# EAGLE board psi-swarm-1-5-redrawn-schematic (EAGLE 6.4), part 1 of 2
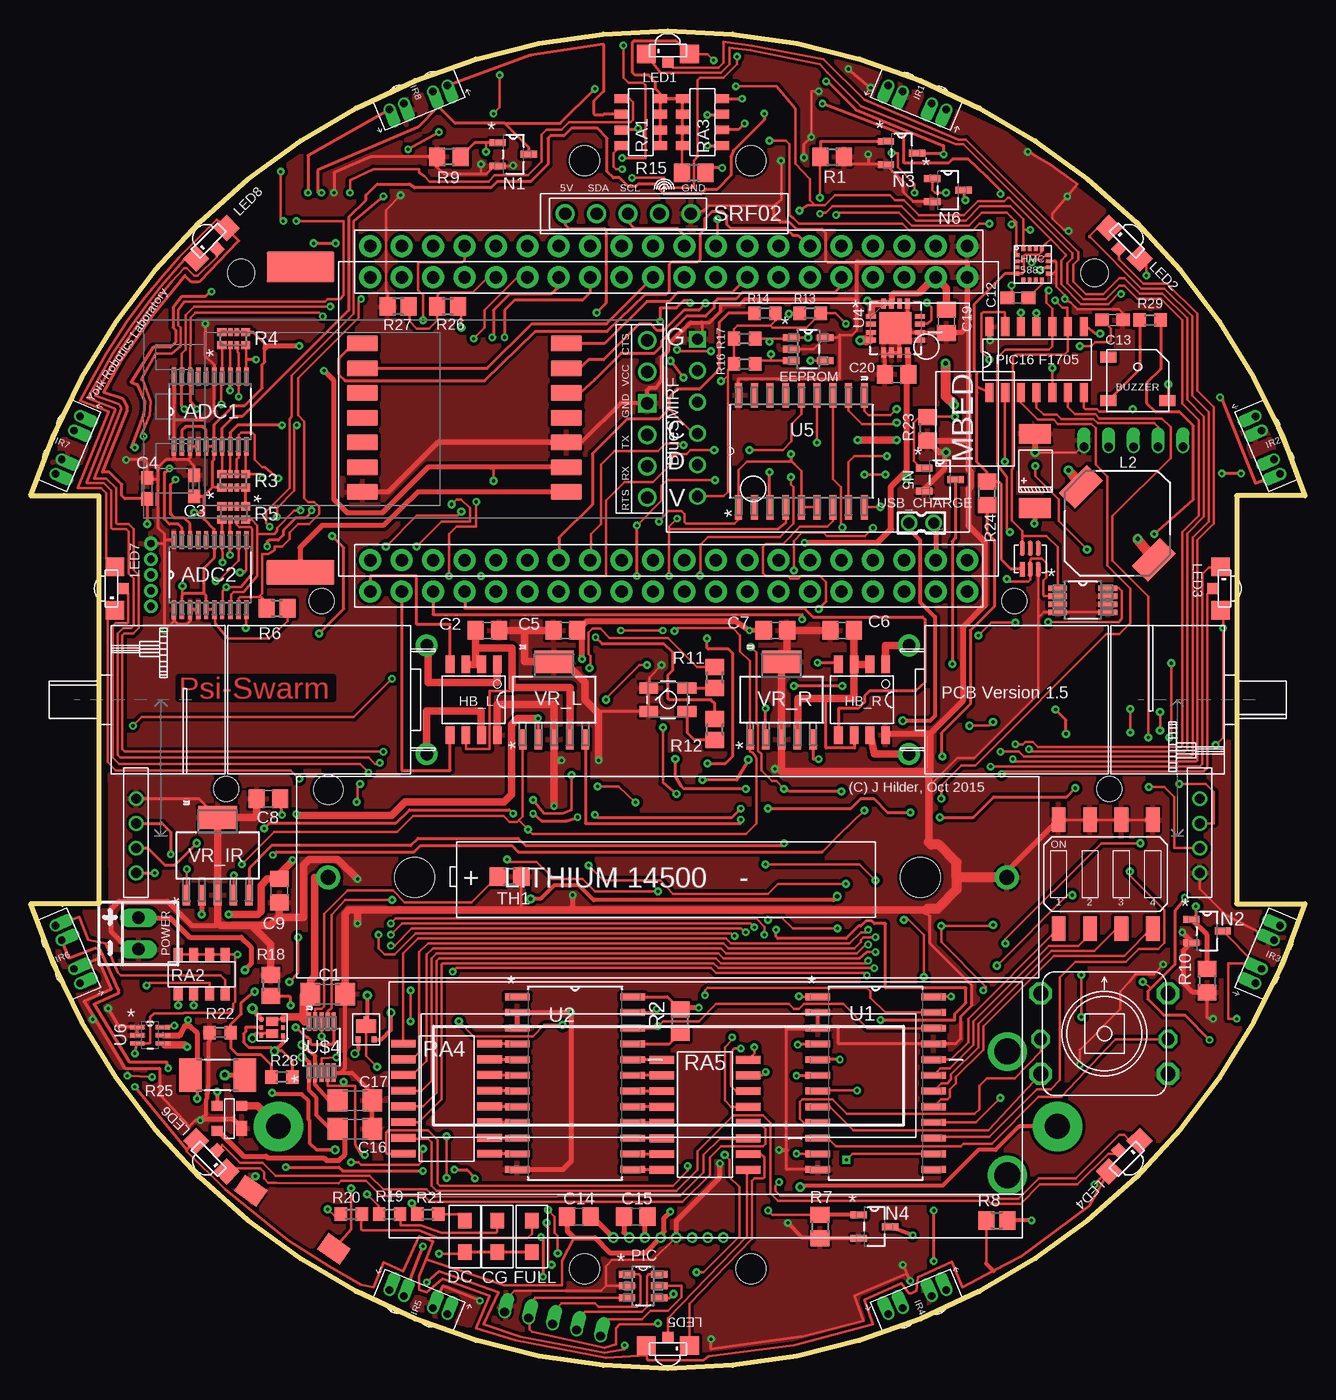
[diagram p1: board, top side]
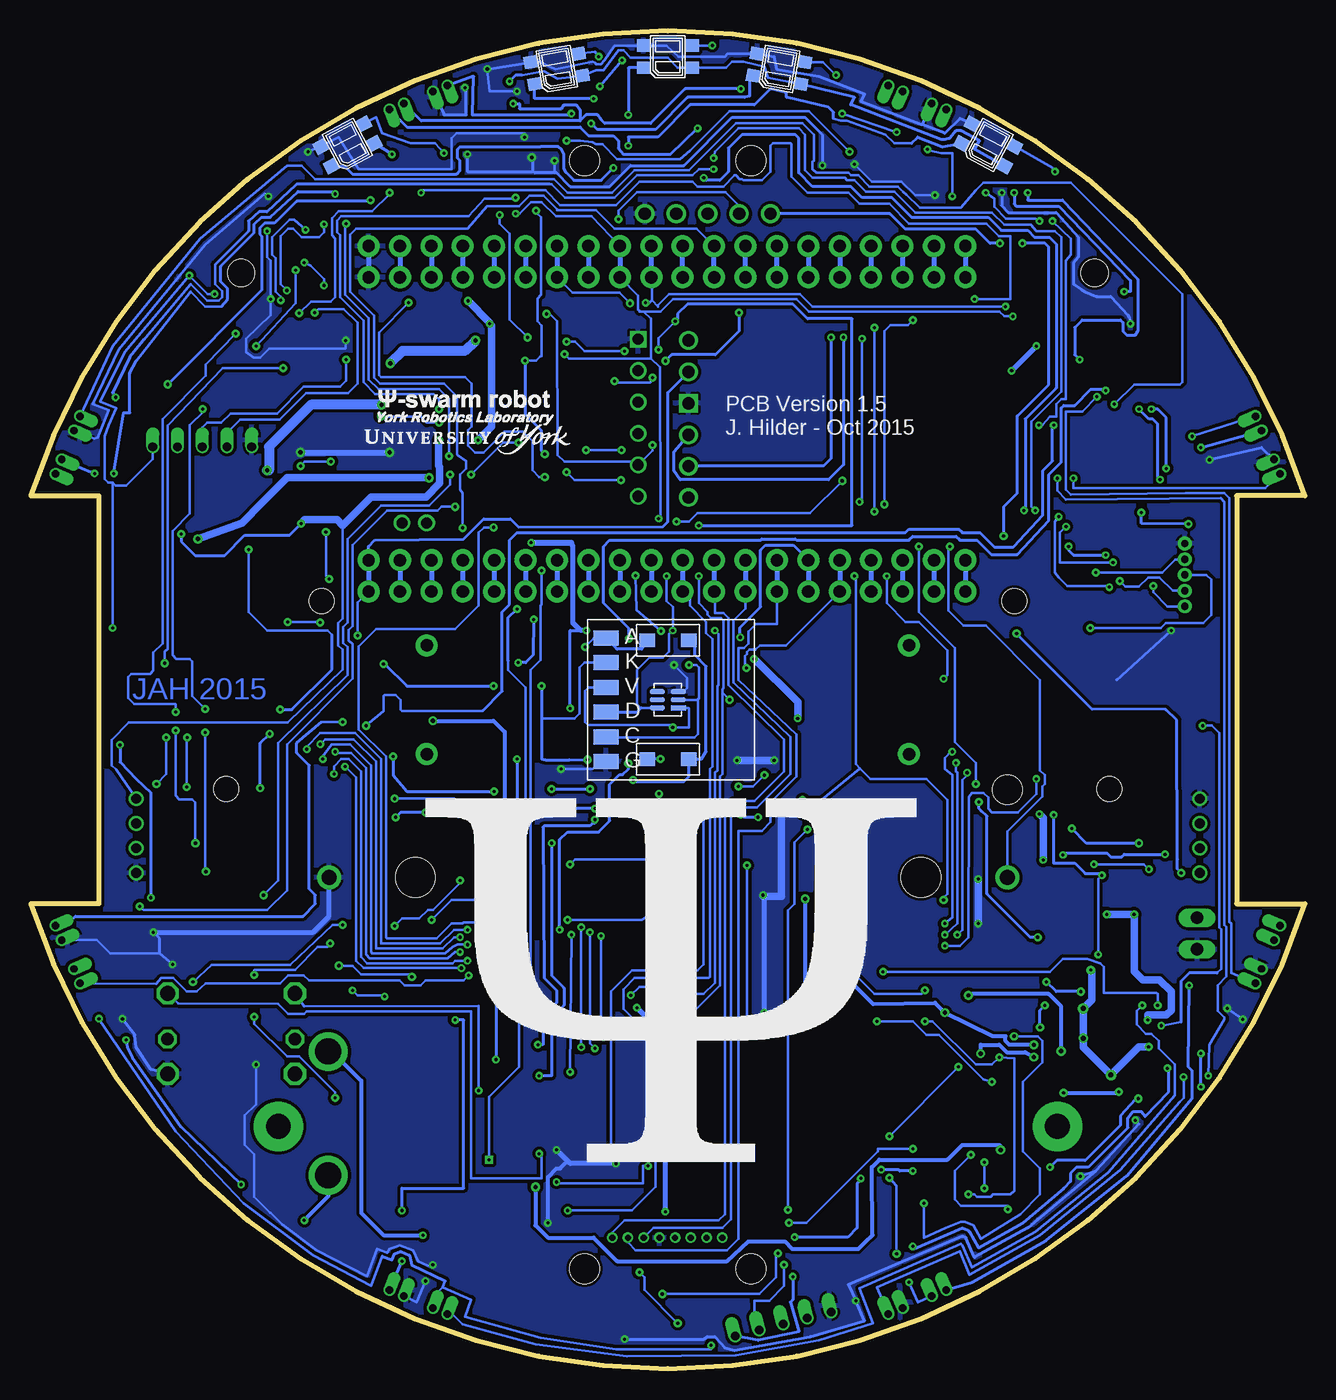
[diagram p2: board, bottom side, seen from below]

Size 103 x 108.16 mm. Coordinates in mm from the lower left corner, seen from the top.
Outline: 0,70.58 arc-144 103,70.58 97.5,70.58 97.5,37.58 103,37.58 arc-144 0,37.58 5.5,37.58 5.5,70.58 0,70.58
Copper layers (1*16): Top 0.018mm / dielectric 1.55mm / Bottom 0.018mm
Design rules "eC_2Layer_PClass6_BaseCopperO18_eCDefault *": minimum track width 0.15mm, minimum drill 0.25mm, track to track 0.15mm, track to pad 0.15mm, pad to pad 0.15mm, via to via 0.15mm, smd to smd 0mil, copper to edge 0.25mm, drill to drill 0.25mm, minimum pad ring 0.175mm, minimum via ring 0.125mm, stop-mask expansion 0mil, vias tented up to drill 0.45mm, thermal gap 0.2mm
Holes 2.4 mm at 44.77,97.68 58.23,97.68 44.77,8.08 58.23,8.08
Holes 2.2 mm at 17,88.58 86,88.58
Holes 2 mm at 23.5,62.08 79.5,62.08 15.8,46.88 87.2,46.88

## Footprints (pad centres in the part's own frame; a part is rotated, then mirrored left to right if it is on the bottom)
SOP65P640X120-20N = smd 1.473 x 0.356: 1 -2.819,2.921; 2 -2.819,2.286; 3 -2.819,1.626; 4 -2.819,0.965; 5 -2.819,0.33; 6 -2.819,-0.33; 7 -2.819,-0.965; 8 -2.819,-1.626; 9 -2.819,-2.286; 10 -2.819,-2.921; 11 2.819,-2.921; 12 2.819,-2.286; 13 2.819,-1.626; 14 2.819,-0.965; 15 2.819,-0.33; 16 2.819,0.33; 17 2.819,0.965; 18 2.819,1.626; 19 2.819,2.286; 20 2.819,2.921
C1206 = smd 1.6 x 1.8: 1 -1.4,0; 2 1.4,0
C0805 = smd 1.3 x 1.5: 1 -0.95,0; 2 0.95,0
C0603 = smd 1.1 x 1: 1 -0.85,0; 2 0.85,0
2917TANTALUM = smd 1.6 x 2.6: ANODE -3,0; CATHODE 3,0
SOT95P270X145-5N = smd 1.321 x 0.559: 1 -1.372,0.94; 2 -1.372,0; 3 -1.372,-0.94; 4 1.372,-0.94; 5 1.372,0.94
ROHM-BD6211 = smd 0.7 x 1.4: P$1 -1.905,-2.857; P$2 -0.635,-2.857; P$3 0.635,-2.857; P$4 1.905,-2.857; P$5 1.905,2.857; P$6 0.635,2.857; P$7 -0.635,2.857; P$8 -1.905,2.857
TCRT-1000 = drill 0.6 pad 1.016 offset: ANODE -2.54,1.2; CATHODE -1.27,1.2; COLLECTOR 2.54,1.2; EMITTER 1.27,1.2
QRE1113GR-1471020 = smd 1.1 x 1: P1-ANODE -1.95,-0.9; P2-CATHODE 1.95,-0.9; P3-COLLECTOR 1.95,0.9; P4-EMITTER -1.95,0.9
IND_ELL8TP = smd 1.8 x 3.2 rotated 45: 1 -2.95,-2.95; 2 2.95,2.95
KINGBRIGHT-KPBA3010 = smd 1.5 x 1.5: P1-ANODE -1.75,1.8; P3-CGREEN 1.75,1.8 | smd 0.9 x 0.9: P2-CRED 0,2.45
2322113-DUAL-LED-WURTH1411 = smd 1.5 x 0.9: 1 1.55,0.95; 2 1.55,-0.95; 3 -1.55,0.95; 4 -1.55,-0.95
01-ROBOT_LED-SMD = smd 1.25 x 1.1: AN -1.675,0; CA 1.675,0
MICROMETALGEARMOTOR = drill 1 pad 1.778: MOTOR+ 25.5,4.4; MOTOR- 25.5,-4.4
01-ROBOT_SOT95P280X130-3N = smd 1.321 x 0.559: 1 -1.27,0.94; 2 -1.27,-0.94; 3 1.27,0
01-ROBOT_SOT95P270X145-6N = smd 1.321 x 0.559: 1 -1.295,0.94; 2 -1.295,0; 3 -1.295,-0.94; 4 1.295,-0.94; 5 1.295,0; 6 1.295,0.94
22-23-2021 = drill 1 long: 1 -1.27,0; 2 1.27,0
R0805 = smd 1.3 x 1.5: 1 -0.95,0; 2 0.95,0
RESCAXE50P210X110X45-8N = smd 0.66 x 0.762: 1 -0.533,0.965; 4 -0.533,-0.965; 5 0.533,-0.965; 8 0.533,0.965 | smd 0.66 x 0.356: 2 -0.533,0.254; 3 -0.533,-0.254; 6 0.533,-0.254; 7 0.533,0.254
R0805' = smd 1.3 x 1.5: 1 -0.85,0; 2 0.85,0
R0603 = smd 1 x 1.1: 1 -0.85,0; 2 0.85,0
R2010 = smd 1.8 x 2.7: 1 -2.2,0; 2 2.2,0
VISHAY-CRA12E083-RES_ARRAY = smd 0.72 x 1.05: 1A 0,-1.6; 1B 0,1.6; 2A 1.27,-1.6; 2B 1.27,1.6; 3A 2.54,-1.6; 3B 2.54,1.6; 4A 3.81,-1.6; 4B 3.81,1.6
BOURNS-4816P = smd 2 x 0.63: 1 -3.493,0; 2 -3.493,-1.27; 3 -3.493,-2.54; 4 -3.493,-3.81; 5 -3.493,-5.08; 6 -3.493,-6.35; 7 -3.493,-7.62; 8 -3.493,-8.89; 9 3.493,-8.89; 10 3.493,-7.62; 11 3.493,-6.35; 12 3.493,-5.08; 13 3.493,-3.81; 14 3.493,-2.54; 15 3.493,-1.27; 16 3.493,0
ALPS-SKQUCAA010 = drill 1.2 octagon: P1 -5.15,3.25; P3 -5.15,-3.25; P4 5.15,-3.25; P6 5.15,3.25 | drill 1 octagon: P2 -5.15,-0.45; P5 5.15,-0.45
4WAYDIL-MCEMR-04-T = smd 1.1 x 2: 1 -3.81,-4.4; 2 -1.27,-4.4; 3 1.27,-4.4; 4 3.81,-4.4; 5 3.81,4.4; 6 1.27,4.4; 7 -1.27,4.4; 8 -3.81,4.4
SWITCH-1703878 = smd 2.2 x 1.6: 1 0,0; 2 8.2,0
01-ROBOT_SOIC127P1030X265-24N = smd 1.981 x 0.559: 1 -4.674,6.985; 2 -4.674,5.715; 3 -4.674,4.445; 4 -4.674,3.175; 5 -4.674,1.905; 6 -4.674,0.635; 7 -4.674,-0.635; 8 -4.674,-1.905; 9 -4.674,-3.175; 10 -4.674,-4.445; 11 -4.674,-5.715; 12 -4.674,-6.985; 13 4.674,-6.985; 14 4.674,-5.715; 15 4.674,-4.445; 16 4.674,-3.175; 17 4.674,-1.905; 18 4.674,-0.635; 19 4.674,0.635; 20 4.674,1.905; 21 4.674,3.175; 22 4.674,4.445; 23 4.674,5.715; 24 4.674,6.985
QFN65P400X400X100-17N = smd 0.813 x 0.381: 1 -1.981,0.965; 2 -1.981,0.33; 3 -1.981,-0.33; 4 -1.981,-0.965; 9 1.981,-0.965; 10 1.981,-0.33; 11 1.981,0.33; 12 1.981,0.965 | smd 0.381 x 0.813: 5 -0.965,-1.981; 6 -0.33,-1.981; 7 0.33,-1.981; 8 0.965,-1.981; 13 0.965,1.981; 14 0.33,1.981; 15 -0.33,1.981; 16 -0.965,1.981 | smd 2.591 x 2.591: 17 0,0
01-ROBOT_SOIC127P1030X265-18N = smd 1.981 x 0.559: 1 -4.521,5.08; 2 -4.521,3.81; 3 -4.521,2.54; 4 -4.521,1.27; 5 -4.521,0; 6 -4.521,-1.27; 7 -4.521,-2.54; 8 -4.521,-3.81; 9 -4.521,-5.08; 10 4.521,-5.08; 11 4.521,-3.81; 12 4.521,-2.54; 13 4.521,-1.27; 14 4.521,0; 15 4.521,1.27; 16 4.521,2.54; 17 4.521,3.81; 18 4.521,5.08
4WHEEL_ROBOT_LIBRARY_SOT65P210X110-6N = smd 1.168 x 0.356: 1 -1.041,0.66; 2 -1.041,0; 3 -1.041,-0.66; 4 1.041,-0.66; 5 1.041,0; 6 1.041,0.66
01-ROBOT_MBED-DUALSOCKET = drill 1 pad 1.778: P$1 0,0; P$2 0,-2.54; P$3 0,-5.08; P$4 0,-7.62; P$5 0,-10.16; P$6 0,-12.7; P$7 0,-15.24; P$8 0,-17.78; P$9 0,-20.32; P$10 0,-22.86; P$11 0,-25.4; P$12 0,-27.94; P$13 0,-30.48; P$14 0,-33.02; P$15 0,-35.56; P$16 0,-38.1; P$17 0,-40.64; P$18 0,-43.18; P$19 0,-45.72; P$20 0,-48.26; P$21 22.86,-48.26; P$22 22.86,-45.72; P$23 22.86,-43.18; P$24 22.86,-40.64; P$25 22.86,-38.1; P$26 22.86,-35.56; P$27 22.86,-33.02; P$28 22.86,-30.48; P$29 22.86,-27.94; P$30 22.86,-25.4; P$31 22.86,-22.86; P$32 22.86,-20.32; P$33 22.86,-17.78; P$34 22.86,-15.24; P$35 22.86,-12.7; P$36 22.86,-10.16; P$37 22.86,-7.62; P$38 22.86,-5.08; P$39 22.86,-2.54; P$40 22.86,0; P$41 -2.54,0; P$42 -2.54,-2.54; P$43 -2.54,-5.08; P$44 -2.54,-7.62; P$45 -2.54,-10.16; P$46 -2.54,-12.7; P$47 -2.54,-15.24; P$48 -2.54,-17.78; P$49 -2.54,-20.32; P$50 -2.54,-22.86; P$51 -2.54,-25.4; P$52 -2.54,-27.94; P$53 -2.54,-30.48; P$54 -2.54,-33.02; P$55 -2.54,-35.56; P$56 -2.54,-38.1; P$57 -2.54,-40.64; P$58 -2.54,-43.18; P$59 -2.54,-45.72; P$60 -2.54,-48.26; P$61 25.4,-48.26; P$62 25.4,-45.72; P$63 25.4,-43.18; P$64 25.4,-40.64; P$65 25.4,-38.1; P$66 25.4,-35.56; P$67 25.4,-33.02; P$68 25.4,-30.48; P$69 25.4,-27.94; P$70 25.4,-25.4; P$71 25.4,-22.86; P$72 25.4,-20.32; P$73 25.4,-17.78; P$74 25.4,-15.24; P$75 25.4,-12.7; P$76 25.4,-10.16; P$77 25.4,-7.62; P$78 25.4,-5.08; P$79 25.4,-2.54; P$80 25.4,0
KEYSTONE-1028-AAHOLDER = drill 1.2 pad 1.93: + 2.54,8.13; - 57.4,8.13 | hole 3.2: 9.53,8.13; 50.41,8.13 | hole 2.38: 2.54,15.22
01-ROBOT_MIDAS-MCCOG21605B6W-DISPLAY = drill 0.5: 1-VOUT 18.155,0; 2-CAPN 19.425,0; 3-CAPP 20.695,0; 4-VDD 21.965,0; 5-VSS 23.235,0; 6-SDA 24.505,0; 7-SCL 25.775,0; 8-RST 27.045,0 | drill 2.1: LED-A 50,5.05; LED-K 50,15.05
01-ROBOT_SOP50P490X110-8N = smd 1.499 x 0.33: 1 -2.057,0.991; 2 -2.057,0.508; 3 -2.057,0; 4 -2.057,-0.508; 5 -2.057,-0.991; 6 2.057,-0.991; 7 2.057,-0.508; 8 2.057,0; 9 2.057,0.508; 10 2.057,0.991
HMC5883L = smd 0.45 x 0.3: P$1 -1.3,0.75; P$2 -1.3,0.25; P$3 -1.3,-0.25; P$4 -1.3,-0.75; P$9 1.3,-0.75; P$10 1.3,-0.25; P$11 1.3,0.25; P$12 1.3,0.75 | smd 0.3 x 0.45: P$5 -0.75,-1.3; P$6 -0.25,-1.3; P$7 0.25,-1.3; P$8 0.75,-1.3; P$13 0.75,1.3; P$14 0.25,1.3; P$15 -0.25,1.3; P$16 -0.75,1.3
POLOLU_LIBRARY_ALPHA433 = smd 1.3 x 2.5: 1-SDO 0,0; 2-NIRQ 2,0; 3-FSK 4,0; 4-DCLK 6,0; 5-CLK 8,0; 6-NRES 10,0; 7-GND 12,0; 8-ANT 12,16.5; 9-VDD 10,16.5; 10-GND 8,16.5; 11-NINT 6,16.5; 12-SDI 4,16.5; 13-SCLK 2,16.5; 14-NSEL 0,16.5
NEW_PSISWARM_LIBRARY_PIC16F1705 = smd 0.65 x 1.55: P$1 0,-2.667; P$2 1.27,-2.667; P$3 2.54,-2.667; P$4 3.81,-2.667; P$5 5.08,-2.667; P$6 6.35,-2.667; P$7 7.62,-2.667; P$8 7.62,2.667; P$9 6.35,2.667; P$10 5.08,2.667; P$11 3.81,2.667; P$12 2.54,2.667; P$13 1.27,2.667; P$14 0,2.667
POLOLU_LIBRARY_2148530-433MHZANTENNA = smd 5.5 x 2: ANT 0,0 | smd 5.5 x 2.5: NC 0,24.7
NEW_PSISWARM_LIBRARY_SRF02-MODULE = drill 1 pad 1.55: 1-5V 0,0; 2-SDA 2.54,0; 3-SCL 5.08,0; 4-NC 7.62,0; 5-GND 10.16,0
01-ROBOT_BLUESMIRF-MODULE = drill 1: CTS -1.27,6.35; RTS -1.27,-6.35; RX -1.27,-3.81; TX -1.27,-1.27; VCC -1.27,3.81 | drill 1 square: GND -1.27,1.27
01-ROBOT_PMEG2020CPA-CCDIODE-1859909 = smd 0.4 x 0.5: P$1 -0.65,1.05; P$2 0.65,1.05 | smd 1.6 x 1.1: P$3 0,0 | smd 0.4 x 0.25: P$4 0,-0.675
EXPORTED_LIBRARYPSI-SWARM-V13_01-ROBOT_LED-SMD = smd 1.25 x 1.1: AN -1.275,0; CA 1.275,0
2191755-PMFPB8032XP-MOSFET-SCHOTTKY = smd 0.35 x 0.3: 1 -0.65,-0.875; 2 0,-0.875; 3 0.65,-0.875; 4 0.65,0.875; 5 0,0.875; 6 -0.65,0.875 | smd 0.7 x 1: 7 -0.49,0; 8 0.49,0
EXPORTED_LIBRARYPSI-SWARM-V13_01-ROBOT_P-TERMINALS = drill 2 pad 4: P$1 3,0; P$2 66,0
01-ROBOT_1791469-SCHOTTKY-BRIDGE = smd 1.2 x 0.9: 1 -0.8,-1 | smd 0.8 x 0.9: 2 1,-1; 3 1,1; 4 -1,1
TCS34725FNCOLOURSENSOR = smd 1.2 x 0.4: 1-VDD -0.85,0.65; 2-SCL -0.85,0; 3-GND -0.85,-0.65; 4-NC 0.85,-0.65; 5-INT 0.85,0; 6-SDA 0.85,0.65
5-PIN-2MM = drill 0.7 offset: 1 0,0; 2 2,0; 3 4,0; 4 6,0; 5 8,0
WHEEL-ENCODER = drill 0.8: CHA 0,1; CHB 0,-1; GND 0,3; VCC-5V 0,-3
WHEEL-ENCODER-RIGHT = drill 0.8: CHA 0,-1; CHB 0,1; GND 0,-3; VCC-5V 0,3
POLOLU_LIBRARY_SOP65P490X110-8N = smd 1.524 x 0.457: 1 -2.032,0.965; 2 -2.032,0.33; 3 -2.032,-0.33; 4 -2.032,-0.965; 5 2.032,-0.965; 6 2.032,-0.33; 7 2.032,0.33; 8 2.032,0.965
SMT-0540-T-2-RBUZZER = smd 1.3 x 0.9: + 0.1,0.9; - 4.9,0.9; DUMMY 0.1,4.4
1.27MMPITCH5PIN = drill 0.6 pad 1.1: P$1 0,0; P$2 0,1.27; P$3 0,2.54; P$4 0,3.81; P$5 0,5.08
COLOUR_SENSOR_MODULE = smd 2 x 1.2: GND -5,-5; LED_A -5,5; LED_K -5,3; SCL -5,-3; SDA -5,-1; VDD -5,1
TILT-COMP-COMPASS-MODULE = drill 0.9: 5V 2.5,2.9; -MODE 2.5,10.52; -NC 2.5,13.06; SCL 2.5,7.98; SDA 2.5,5.44 | drill 0.9 square: GND 2.5,15.6
87758-0216 = drill 0.9 pad 1.27: 1 0,-1; 2 0,1
01-ROBOT_SOT230P700X180-6N = smd 1.626 x 0.61: 1 -3.2,2.54; 2 -3.2,1.27; 3 -3.2,0; 4 -3.2,-1.27; 5 -3.2,-2.54 | smd 1.854 x 3.175: 6 3.073,0

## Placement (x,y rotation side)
ADC1  AD7997BRUZ-1  [SOP65P640X120-20N]  14.5,77.38 90 top
ADC2  AD7997BRUZ-1  [SOP65P640X120-20N]  14.5,64.18 90 top
C1  4.7u  [C1206]  24,30.28 0 top
C2  4.7u  [C0805]  36.9,59.68 0 top
C3  1u  [C0603]  13.2,71.38 90 top
C4  100n  [C0603]  9.4,71.18 90 top
C5  4.7u  [C0805]  43.2,59.68 180 top
C6  4.7u  [C0805]  65.6,59.68 180 top
C7  4.7u  [C0805]  60.2,59.68 0 top
C8  4.7u  [C0805]  19.2,46.08 180 top
C9  4.7u  [C0805]  20.1,38.63 270 top
C12  220N  [C0603]  79.8,86.58 0 top
C13  4.7U  [C0603]  87.45,84.78 180 top
C14  4.7u  [C0805]  44.3,12.28 180 top
C15  4.7u  [C0805]  48.9,12.28 0 top
C16  4.7u  [C1206]  26.2,19.38 0 top
C17  4.7u  [C1206]  26.2,21.68 0 top
C18  150uF TANT  [2917TANTALUM]  81.17,72.58 90 top
C19  2.2uF  [C0805]  74.02,84.68 270 top
C20  10uF  [C0805]  69.99,80.4 0 top
EEPROM  24AA64T-I/OT  [SOT95P270X145-5N]  62.85,82.43 0 top
HB_L  HBRIDGE-BD6211FE2-1716259  [ROHM-BD6211]  35.8,54.08 180 top
HB_R  HBRIDGE-BD6211FE2-1716259  [ROHM-BD6211]  67.2,54.08 180 top
IR1  TCRT-1000  [TCRT-1000]  72.13,103.88 157.5 top
IR2  TCRT-1000  [TCRT-1000]  101.11,75.14 113 top
IR3  TCRT-1000  [TCRT-1000]  101.11,33.02 67 top
IR4  TCRT-1000  [TCRT-1000]  72.13,4.28 22.5 top
IR5  TCRT-1000  [TCRT-1000]  30.87,4.28 337.5 top
IR6  TCRT-1000  [TCRT-1000]  1.88,33.02 293 top
IR7  TCRT-1000  [TCRT-1000]  1.88,75.14 247 top
IR8  TCRT-1000  [TCRT-1000]  30.87,103.88 202.5 top
IR_B1  QRE1113GR-1471020  [QRE1113GR-1471020]  25.6,98.94 332 bottom
IR_B2  QRE1113GR-1471020  [QRE1113GR-1471020]  42.51,105.09 350 bottom
IR_B3  QRE1113GR-1471020  [QRE1113GR-1471020]  51.5,106.08 0 bottom
IR_B4  QRE1113GR-1471020  [QRE1113GR-1471020]  60.49,105.09 10 bottom
IR_B5  QRE1113GR-1471020  [QRE1113GR-1471020]  77.4,98.94 28 bottom
L2  6.8UH  [IND_ELL8TP]  87.85,68.35 270 top
LED1  KPBA3010-DUAL-LED  [KINGBRIGHT-KPBA3010]  51.5,108.08 180 top
LED2  KPBA3010-DUAL-LED  [KINGBRIGHT-KPBA3010]  89.68,92.26 135 top
LED3  KPBA3010-DUAL-LED  [KINGBRIGHT-KPBA3010]  98,63.08 90 top
LED4  KPBA3010-DUAL-LED  [KINGBRIGHT-KPBA3010]  89.68,15.9 45 top
LED5  KPBA3010-DUAL-LED  [KINGBRIGHT-KPBA3010]  51.5,0.08 0 top
LED6  KPBA3010-DUAL-LED  [KINGBRIGHT-KPBA3010]  13.32,15.9 315 top
LED7  KPBA3010-DUAL-LED  [KINGBRIGHT-KPBA3010]  5,63.08 270 top
LED8  KPBA3010-DUAL-LED  [KINGBRIGHT-KPBA3010]  13.32,92.26 225 top
LED9  2322113-WURTH-DUALLED  [2322113-DUAL-LED-WURTH1411]  51.5,54.08 0 top
LED10  01-ROBOT_KINGBRIGHT-KP-2012-2290331-2335811-2335796  [01-ROBOT_LED-SMD]  51.5,58.88 0 bottom
LED11  01-ROBOT_KINGBRIGHT-KP-2012-2290331-2335811-2335796  [01-ROBOT_LED-SMD]  51.5,49.28 0 bottom
LEFT_MOTOR  MICROMETALGEARMOTOR12MM  [MICROMETALGEARMOTOR]  6.5,54.08 0 top
N1  01-ROBOT_TSM2310CX  [01-ROBOT_SOT95P280X130-3N]  39,98.18 0 top
N2  01-ROBOT_TSM2310CX  [01-ROBOT_SOT95P280X130-3N]  95.1,35.38 0 top
N3  01-ROBOT_TSM2310CX  [01-ROBOT_SOT95P280X130-3N]  70.4,98.28 0 top
N4  01-ROBOT_TSM2310CX  [01-ROBOT_SOT95P280X130-3N]  68.2,11.48 0 top
N5  01-ROBOT_TSM2310CX  [01-ROBOT_SOT95P280X130-3N]  73.5,71.88 0 top
N6  01-ROBOT_TSM2310CX  [01-ROBOT_SOT95P280X130-3N]  74.15,95.28 0 top
PIC  01-ROBOT_PIC10F202T-I/OT  [01-ROBOT_SOT95P270X145-6N]  49.5,6.68 0 top
POWER  ALT.Power.In  [22-23-2021]  8.7,35.18 90 top
R1  100K  [R0805]  64.8,97.98 0 top
R2  10k  [R0805]  52.5,28.08 90 top
R3  10K  [RESCAXE50P210X110X45-8N]  16.4,71.78 90 top
R4  10K  [RESCAXE50P210X110X45-8N]  16.4,83.28 90 top
R5  10K  [RESCAXE50P210X110X45-8N]  16.4,69.18 270 top
R6  10k  [R0805']  19.9,61.48 0 top
R7  100K  [R0805]  63.8,11.48 270 top
R8  68  [R0805']  78.1,11.98 0 top
R9  100K  [R0805]  33.8,97.98 180 top
R10  100K  [R0805]  95.1,31.38 270 top
R11  100  [R0805']  55.3,55.88 90 top
R12  100  [R0805']  55.3,51.68 90 top
R13  2K2  [R0603]  63,85.33 0 top
R14  2K2  [R0603]  59.35,85.33 0 top
R15  22  [R0805]  53.6,96.68 180 top
R16  2K2  [R0603]  57.7,81.23 0 top
R17  2K2  [R0603]  57.7,83.28 0 top
R18  3k3 for 300ma chg  [R0805']  19.4,30.98 270 top
R19  2k2  [R0603]  29,12.48 180 top
R20  2k2  [R0603]  25.9,12.48 180 top
R21  2k2  [R0603]  32.1,12.48 180 top
R22  47k  [R0603]  15.3,27.18 0 top
R23  100K  [R0805]  72.5,75.98 270 top
R24  47  [R0805]  77.3,70.78 90 top
R25  [R2010]  15.09,23.73 180 top
R26  100k  [R0805']  33.7,85.88 0 top
R27  200k  [R0805']  29.7,85.88 180 top
R28  47k  [R0603]  20.3,23.58 0 top
R29  [R0603]  90.5,84.78 0 top
RA1  22OHM  [VISHAY-CRA12E083-RES_ARRAY]  49.3,102.68 270 top
RA2  22OHM  [VISHAY-CRA12E083-RES_ARRAY]  11.9,31.88 0 top
RA3  22OHM  [VISHAY-CRA12E083-RES_ARRAY]  54.3,98.88 90 top
RA4  100  [BOURNS-4816P]  33.6,26.28 0 top
RA5  100  [BOURNS-4816P]  54.5,16.08 180 top
RIGHT_MOTOR  MICROMETALGEARMOTOR12MM  [MICROMETALGEARMOTOR]  96.5,54.08 180 top
SW1  5-WAY-SWITCH  [ALPS-SKQUCAA010]  86.8,27.08 0 top
SW2  4-WAY-DIP-1524007-MCEMR-04-T  [4WAYDIL-MCEMR-04-T]  86.9,39.98 0 top
SW3  1703878-SWITCH  [SWITCH-1703878]  24.5,9.68 145 top
TH1  10KNTC  [R0805]  38.7,39.78 180 top
U1  PCA9555  [01-ROBOT_SOIC127P1030X265-24N]  68.3,23.08 0 top
U2  PCA9555  [01-ROBOT_SOIC127P1030X265-24N]  44,23.08 0 top
U4  TPS61032RSAR  [QFN65P400X400X100-17N]  69.91,84.12 0 top
U5  01-ROBOT_MCP23009-E/SO  [01-ROBOT_SOIC127P1030X265-18N]  62.3,74.18 90 top
U6  INA211  [4WHEEL_ROBOT_LIBRARY_SOT65P210X110-6N]  9.63,26.96 0 top
U$1  01-ROBOT_MBED-LPC1768-DUALSOCKET  [01-ROBOT_MBED-DUALSOCKET]  75.7,88.23 270 top
U$2  AA-14500-KEYSTONE1028-HOLDER  [KEYSTONE-1028-AAHOLDER]  21.5,31.58 0 top
U$3  01-ROBOT_DISPLAY-2218942-MIDAS-MCCOG21605B6W-FPTLWI  [01-ROBOT_MIDAS-MCCOG21605B6W-DISPLAY]  28.95,10.58 0 top
U$4  01-ROBOT_MCP73837-FCI/UN  [01-ROBOT_SOP50P490X110-8N]  23.5,25.98 90 top
U$5  HMC5883L  [HMC5883L]  81,89.28 0 top
U$6  POLOLU_LIBRARY_ALPHA433  [POLOLU_LIBRARY_ALPHA433]  26.8,82.88 270 top
U$7  NEW_PSISWARM_LIBRARY_PIC16F1705  [NEW_PSISWARM_LIBRARY_PIC16F1705]  77.5,81.58 0 top
U$8  POLOLU_LIBRARY_ANTENNA  [POLOLU_LIBRARY_2148530-433MHZANTENNA]  21.8,64.38 0 top
U$9  [NEW_PSISWARM_LIBRARY_SRF02-MODULE]  43.2,93.38 0 top
U$10  01-ROBOT_BLUESMIRF-HOBBYTRONICS  [01-ROBOT_BLUESMIRF-MODULE]  51.1,76.78 0 top
U$11  01-ROBOT_1859909-PMEG2020CPA-CCDIODE  [01-ROBOT_PMEG2020CPA-CCDIODE-1859909]  27.1,27.68 180 top
U$12  EXPORTED_LIBRARYPSI-SWARM-V13_01-ROBOT_KINGBRIGHT-KP-2012-2290331-2335811-2335796  [EXPORTED_LIBRARYPSI-SWARM-V13_01-ROBOT_LED-SMD]  37.7,10.68 90 top
U$13  EXPORTED_LIBRARYPSI-SWARM-V13_01-ROBOT_KINGBRIGHT-KP-2012-2290331-2335811-2335796  [EXPORTED_LIBRARYPSI-SWARM-V13_01-ROBOT_LED-SMD]  40.5,10.68 90 top
U$14  EXPORTED_LIBRARYPSI-SWARM-V13_01-ROBOT_KINGBRIGHT-KP-2012-2290331-2335811-2335796  [EXPORTED_LIBRARYPSI-SWARM-V13_01-ROBOT_LED-SMD]  35.1,10.68 90 top
U$15  2191755-MOSFET-SCHOTTKY  [2191755-PMFPB8032XP-MOSFET-SCHOTTKY]  19.5,27.58 90 top
U$16  EXPORTED_LIBRARYPSI-SWARM-V13_01-ROBOT_POWER-TERMS  [EXPORTED_LIBRARYPSI-SWARM-V13_01-ROBOT_P-TERMINALS]  17,19.58 0 top
U$17  01-ROBOT_1791469-SCHOTTKYBRIDGE  [01-ROBOT_1791469-SCHOTTKY-BRIDGE]  16.05,20.23 90 top
U$18  7857746(RS)-COLOUR-SENSOR  [TCS34725FNCOLOURSENSOR]  51.5,54.08 180 bottom
U$19  5-PIN-CON  [5-PIN-2MM]  38.3,4.58 346 top
U$20  7857746(RS)-COLOUR-SENSOR  [TCS34725FNCOLOURSENSOR]  80.8,65.48 90 top
U$21  WHEEL-ENCODER-LEFT  [WHEEL-ENCODER]  8.5,43.08 0 top
U$22  WHEEL-ENCODER-RIGHT  [WHEEL-ENCODER-RIGHT]  94.5,43.08 0 top
U$23  POLOLU_LIBRARY_MCP9808-E/MS  [POLOLU_LIBRARY_SOP65P490X110-8N]  85.05,62.13 0 top
U$24  SMT-0540-T-2-R-BUZZERSMT  [SMT-0540-T-2-RBUZZER]  87,77.38 0 top
U$25  5-PIN-0.5PITCH  [1.27MMPITCH5PIN]  9.7,61.63 0 top
U$26  COLOUR_SENSOR_CONNECTOR  [COLOUR_SENSOR_MODULE]  51.5,54.08 0 bottom
U$27  5-PIN-CON  [5-PIN-2MM]  85.15,74.53 0 top
U$28  CMPS11-TILT-COMP-COMPASS  [TILT-COMP-COMPASS-MODULE]  51.4,67.63 0 top
USB_CHARGE  87758-0216  [87758-0216]  72,68.38 90 top
VR_IR  01-ROBOT_MCP1826T-3302E/DC  [01-ROBOT_SOT230P700X180-6N]  15.1,41.48 90 top
VR_L  01-ROBOT_MCP1826T-3302E/DC  [01-ROBOT_SOT230P700X180-6N]  42.3,54.08 90 top
VR_R  01-ROBOT_MCP1826T-3302E/DC  [01-ROBOT_SOT230P700X180-6N]  60.7,54.08 90 top

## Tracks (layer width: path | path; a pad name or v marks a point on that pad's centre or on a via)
433-CLK  (via drill 0.25 pad 0.65)
  Top 0.254: v54.55,86.13 54,85.58 52.8,85.58 51.2,83.98 50.6,83.98 50.1,84.48 49.2,84.48 46.3,81.58 45.1,81.58 44.4,80.88 U$6.13-SCLK
  Bottom 0.2: v54.55,86.13 55.4,86.98 59.21,86.98 U$1.P$7
  Bottom 0.406: U$1.P$47 U$1.P$7
433-FSS
  Top 0.254: U$1.P$8 57.92,88.2 56.7,86.98 52.3,86.98 51.6,86.28 49.8,86.28 46.4,82.88 U$6.14-NSEL
  Bottom 0.406: U$1.P$48 U$1.P$8
433-INT
  Top 0.254: U$6.2-NIRQ 36.9,80.88 40.5,84.48 46.55,84.48 U$1.P$11
  Bottom 0.406: U$1.P$11 U$1.P$51
433-SDI
  Top 0.254: U$1.P$5 65.54,87.57 64.95,86.98 57.5,86.98 57,86.48 55.5,86.48 55.25,86.23 55.25,85.78 54.55,85.08 53,85.08 51,83.08 51,82.68 50.4,82.08 47.7,82.08 45.6,79.98 44.4,78.88 U$6.12-SDI
  Bottom 0.406: U$1.P$45 U$1.P$5
433-SDO
  Top 0.254: U$6.1-SDO 26.1,82.88 24.9,81.68 24.9,80.38 25.4,79.88 36.7,79.88 40.8,83.88 46.6,83.88 49.7,86.88 51.4,86.88 51.6,87.08 51.6,89.28 51.8,89.48 53.9,89.48 54.1,89.68 54.1,91.78 54.5,92.18 | 61,92.18 61.05,92.18 61.6,91.63 62,91.63 U$1.P$46
  Top 0.256: 54.5,92.18 54.5,92.98 55.1,93.58 55.9,93.58 56.3,93.18 56.3,92.48 56.6,92.18 61,92.18
  Bottom 0.406: U$1.P$46 U$1.P$6
AIN1  (via drill 0.25 pad 0.6)
  Top 0.2: ADC1.7 15.46,72.14 R3.8
  Top 0.254: v59.3,101.48 59.3,100.98 56.8,98.48 56.6,97.98 56.6,96.48 55.5,95.38 54.6,95.38 54.2,94.98 51.2,94.98 50.7,95.48 50.7,95.58 50.5,95.78 49.1,95.78 48.9,95.58 48.3,95.58 47.6,96.28 47.1,96.28 46.6,96.78 46.6,99.48 45.8,100.28 43.7,100.28 43.1,99.68 42,99.68 41.8,99.48 41.8,97.38 40.4,95.98 37.7,95.98 37.2,95.48 31.02,95.48 30.95,95.55 30.6,95.78 28,95.78 27.1,94.88 27.1,94.48 25.7,93.08 25.7,85.58 17.1,76.98 16.4,76.98 15.46,76.04 ADC1.7
  Bottom 0.254: v59.3,101.48 59.4,101.38 67.3,101.38 67.2,104.48 IR1.COLLECTOR
AIN2  (via drill 0.25 pad 0.6)
  Top 0.2: R4.1 15.46,82.71 ADC1.14 15.4,80.13 v15.4,77.98
  Bottom 0.2: IR2.COLLECTOR 96.4,82.68 89.3,91.38 82.3,97.28 81.1,97.28 80,96.18 60.7,96.18 59.6,95.08 56,95.08 54.2,96.88 49.8,96.88 46,100.68 40.6,100.68 39.7,99.78 39.7,97.68 39.8,97.58 39.8,96.98 39.5,96.68 36.9,96.68 36.7,96.48 36.1,96.48 35.2,95.58 32.88,95.58 32.23,94.93 | 15.3,77.88 v15.4,77.98 13.8,79.58 10.1,79.58 9.9,79.78 9.9,86.88 18.9,95.88 26,95.88 26.6,95.28 27.8,93.88 31.1,93.88 32.23,94.93 | 32.5,95.18 32.23,94.93
AIN2_1  (via drill 0.25 pad 0.6)
  Top 0.2: R5.7 16.65,68.22 16.85,68.03 17.75,68.03 17.9,67.88 17.9,64.28 17,63.18 v15.8,63.18 15.5,62.88 15.5,61.39 ADC2.7 | v20.2,96.78 20.2,92.88 v20.4,92.78 | v21.5,76.28 21.3,76.28 21.3,70.98 19.9,69.58 v19.9,68.88
  Bottom 0.2: IR_B1.P3-COLLECTOR 20.4,97.08 v20.2,96.78 | v20.4,92.78 18.9,91.38 18.9,90.08 19.3,89.58 19.3,78.38 19.7,78.38 20.1,77.98 20.1,76.98 20.6,76.98 21.2,76.28 v21.5,76.28 | v19.9,68.88 20.2,68.48 20.2,64.38 19.9,63.98 19.2,63.28 15.8,63.28 v15.8,63.18
AIN2_2  (via drill 0.25 pad 0.6)
  Top 0.2: v37.9,104.58 37.9,101.98 v37.4,101.48 | v33,99.98 v30.5,98.58 | v28.5,94.78 26.1,92.78 26.1,85.28 21.1,80.28 21.1,76.98 20.9,76.78 20.9,71.18 19,69.28 19,68.38 v19.3,68.08 | v15.5,65.18 ADC2.14
  Top 0.254: ADC2.14 15.46,68.61 R5.5
  Bottom 0.2: IR_B2.P3-COLLECTOR 38.96,105.64 v37.9,104.58 | v37.4,101.48 v33,99.98 | v30.5,98.58 30.3,98.48 29.4,98.28 28.5,98.28 v28.5,94.78 | v19.3,68.08 19.8,67.58 19.8,65.18 v15.5,65.18
AIN2_3  (via drill 0.25 pad 0.6)
  Top 0.2: R5.8 17.83,68.65 18.3,68.18 18.3,67.48 | 18.3,67.48 18.3,64.08 17.2,62.78 16.4,62.78 16.2,62.58 16.2,61.43 ADC2.8 | v47.9,106.98 47.9,104.38 48.3,103.98 49.5,103.98 49.7,103.78 49.7,97.88 v47.8,97.88 | v21.8,69.38 21.3,69.38 19.9,67.98 19.9,67.78 19.7,67.48 18.3,67.48
  Bottom 0.2: IR_B3.P3-COLLECTOR v47.9,106.98 | v21.8,69.38 22.1,69.68 22.1,76.58 19.7,78.98 19.7,91.48 20.2,91.98 21.7,91.98 22.15,92.48 24.3,92.48 25.3,93.48 31.5,93.48 33.2,95.18 35.5,95.18 36.4,96.08 37,96.08 37.2,96.28 39.8,96.28 40.4,96.88 40.4,99.78 40.9,100.28 45.8,100.28 47.7,98.38 v47.8,97.88
AIN2_4  (via drill 0.25 pad 0.6)
  Top 0.2: v57.1,106.08 57.1,105.48 56,104.38 54.1,104.38 53.9,104.18 53.9,97.98 53.6,97.68 53.6,95.48 51.4,95.48 51.2,95.68 51.2,96.28 v48.6,96.28
  Top 0.254: R5.6 16.13,68.62 ADC2.13 16.1,66.97 v16.1,65.78 | v22.7,69.38 22.7,69.28 22.2,68.78 21.4,68.78 20.4,67.78 20.4,67.38 20,66.98 19.3,66.98 19.1,66.88 v19.1,66.48
  Bottom 0.2: IR_B4.P3-COLLECTOR 57.4,106.48 v57.1,106.08
  Bottom 0.254: v22.7,69.38 22.6,69.48 22.6,76.78 20.1,79.28 20.1,90.93 20.65,91.48 21.85,91.48 22.4,92.03 24.55,92.03 25.6,93.08 31.8,93.08 33.4,94.68 35.8,94.68 36.7,95.58 39.8,95.58 40.9,96.68 40.9,99.48 41.2,99.78 45.5,99.78 46.6,98.68 46.6,96.78 47.3,96.08 48.4,96.08 v48.6,96.28 | v19.1,66.48 19.1,66.18 18.7,65.78 v16.1,65.78
AIN2_5  (via drill 0.25 pad 0.6)
  Top 0.2: ADC2.9 16.79,62.26 16.9,62.38 18.4,62.38 | 18.4,62.38 18.6,62.38 19.4,61.48 R6.1 | v69.6,98.28 70.1,98.28 70.1,97.13 71.45,95.78 v71.45,95.08 | v26.7,86.48 26.5,86.48 26.5,84.98 21.6,80.08 21.6,77.08 22.1,76.58 22.1,70.38 22.4,70.08 22.9,70.08 23.3,69.68 23.3,69.08 22.5,68.28 21.6,68.28 20.9,67.58 20.9,67.08 20.3,66.48 19.7,66.48 19.7,66.18 19.4,65.98 19.2,65.88 18.7,65.88 18.7,62.68 18.4,62.38
  Bottom 0.2: IR_B5.P3-COLLECTOR 75.1,101.18 74.6,99.88 72.3,99.08 70.3,99.08 v69.6,98.28 | v71.45,95.08 71.45,95.28 61.4,95.28 60.2,94.08 55.7,94.08 53.8,95.98 49.5,95.98 49.1,95.58 47,95.58 46.1,96.48 46,96.48 45.7,96.18 45.5,96.18 45.4,96.08 43.9,96.08 43.2,96.78 43.2,98.88 43,99.08 41.6,99.08 41.5,98.98 41.5,96.38 40.2,95.08 36.9,95.08 36,94.18 33.6,94.18 32,92.58 25.75,92.58 24.75,91.58 23.8,91.58 23.8,86.48 v26.7,86.48
AIN3  (via drill 0.25 pad 0.6, 0.25 pad 0.65)
  Top 0.2: ADC1.8 16.13,72.13 R3.7 | v75.9,51.98 77.5,51.98 v77.8,52.28
  Top 0.254: v20.3,76.28 16.7,76.28 16.1,75.68 16.1,74.58 ADC1.8
  Bottom 0.2: 66.5,53.18 73,53.18 73.1,53.28 73.1,54.08 73.5,54.48 74.4,54.48 74.5,54.38 74.5,53.18 v75.9,51.98 | v77.8,52.28 79.5,52.28
  Bottom 0.254: IR3.COLLECTOR 100.16,35.82 99.4,36.58 81,36.58 80,37.58 80,38.28 80.5,38.78 80.5,48.78 81.5,49.78 81.5,50.58 79.5,52.28 | 66.5,53.18 64.9,54.78 64.9,61.18 64.3,61.78 64.3,66.98 63.7,67.58 32.3,67.58 32,67.88 28,67.88 27.7,67.58 26.25,67.58 25.1,66.43 23.55,66.43 21.2,68.98 21.2,72.58 20.4,73.38 20.4,76.18 v20.3,76.28
AIN4  (via drill 0.25 pad 0.6, 0.25 pad 0.65)
  Top 0.2: ADC1.13 16.13,82.72 R4.2
  Top 0.254: v73,8.68 v73,12.78 | v68.7,28.18 74.7,28.18 74.7,28.68 75.6,29.58 75.6,30.78 69.1,30.78 69.1,35.98 68.2,35.98 68,36.18 67.5,36.18 67.1,35.78 66.9,35.78 65.9,34.78 60.4,34.78 60.25,34.93 v60.25,35.48 | v16.1,79.08 16.1,80.17 ADC1.13 | v54.7,48.93 56.15,48.93 56.75,49.53 56.75,57.83 56.4,58.18 54.75,58.18 54.65,58.28 v54.65,59.03
  Bottom 0.254: IR4.COLLECTOR v73,8.68 | v73,12.78 73,14.58 68,14.58 68,28.18 v68.7,28.18 | v60.25,35.48 60.25,42.78 59.6,43.38 57.1,43.38 56.2,44.28 56.2,47.23 55.4,48.03 55.15,48.03 54.7,48.48 v54.7,48.93 | v16.1,79.08 16.2,79.18 17.3,79.18 18.6,77.88 19.5,77.88 19.7,77.68 19.7,73.28 20.7,72.28 20.7,68.58 23.25,65.83 25.35,65.83 26.5,66.98 27.9,66.98 28.2,67.28 31.7,67.28 32,66.98 41.1,66.98 41.2,67.08 43.9,67.08 44,66.98 56.2,66.98 56.7,66.48 56.7,61.88 54.65,59.83 v54.65,59.03
AIN5  (via drill 0.25 pad 0.6)
  Top 0.2: R3.6 16.65,73.53 16.8,73.68 16.8,73.88 16.8,75.48 17,75.68 17.9,75.68 18.1,75.48 18.1,73.48 18.7,72.88 18.9,72.88 v20,71.98 | v7.8,23.68 v9.8,23.58
  Top 0.254: ADC1.9 16.79,73.89 16.8,73.88
  Bottom 0.2: v20,71.98 20,70.98 19.3,70.28 6.8,70.38 6.5,70.08 6.5,37.98 6.5,37.48 6.5,35.88 6.35,35.73 6.35,31.73 7.05,30.98 7.05,28.93 6.5,28.38 6.5,28.23 7.7,26.18 v7.8,23.68 | v9.8,23.58 9.8,21.88 10.1,21.58 14.9,16.08 21.4,10.78 27.1,7.58 27.9,9.48 34.6,6.58 IR5.COLLECTOR
AIN6  (via drill 0.25 pad 0.6)
  Top 0.2: R4.3 16.7,82.7 16.7,82.18 16.79,82.09 ADC1.12 16.8,80.18 v16.8,78.58
  Bottom 0.2: IR6.COLLECTOR 4.44,31.34 5.95,31.98 5.95,35.98 6.1,36.13 6.1,37.83 6.1,38.18 6.1,70.38 6.5,70.78 9.6,70.78 18.9,70.68 19.3,71.08 19.3,77.38 18,77.38 v16.8,78.58
AIN7  (via drill 0.25 pad 0.6)
  Top 0.2: ADC1.10 17.36,74.5 R3.5 18.57,72.31 18.7,72.18 v18.7,71.98
  Bottom 0.2: v18.7,71.98 18.7,71.18 3.2,71.18 IR7.COLLECTOR
AIN8  (via drill 0.25 pad 0.6)
  Top 0.2: ADC1.11 17.42,81.58 17.42,82.69 R4.4
  Top 0.254: IR8.COLLECTOR 22.4,98.08 v22.4,95.08 | v18.2,81.58 17.42,81.58
  Bottom 0.254: v22.4,95.08 22.4,94.48 19.6,94.48 13.5,88.08 13.5,83.88 13.7,83.58 14.4,83.58 14.7,83.88 14.7,84.58 14.9,84.78 18,84.78 18.6,84.18 18.6,81.98 v18.2,81.58
AUX_INT  (via drill 0.25 pad 0.65)
  Top 0.2: U1.14 66.44,17.36 v65.95,16.88 | 64.3,62.03 64.3,63.58 63.8,64.08 62.25,64.08 62.05,63.88 61.4,63.88 61.2,64.08 59.45,64.08 59.2,64.33 59.2,66.43 59.45,66.68 60.8,66.68 62.2,68.08 64.4,68.08 64.85,68.53 U5.7
  Top 0.256: v63.7,61.43 64.3,62.03
  Bottom 0.2: v65.95,16.88 65.95,21.98 63.55,24.38 63.55,30.48 63,31.03 63,55.08 64.4,56.48 64.4,57.23
  Bottom 0.256: 64.4,57.23 64.4,60.73 v63.7,61.43
B_BLUE  (via drill 0.25 pad 0.65)
  Top 0.2: ADC2.11 17.42,64.55 17.25,64.38 v16.9,64.38
  Bottom 0.2: v16.9,64.38 11.5,64.38 10.45,65.43 U$25.P$4
B_GREEN  (via drill 0.25 pad 0.65)
  Top 0.2: ADC2.10 17.4,61.36 17.4,59.93 v17.35,59.88
  Bottom 0.2: v17.35,59.88 11.65,59.88 11.25,60.28 8.2,60.28 7.55,60.93 7.55,63.78 7.95,64.18 U$25.P$3
B_LED_A  (via drill 0.25 pad 0.65)
  Top 0.2: v58.2,58.33 58.65,57.88 58.65,52.18 58.8,52.03 58.8,49.93 59.05,49.68 59.05,48.36 59.92,47.49 60.28,47.49 v60.9,46.88
  Top 0.254: R24.1 77.3,67.58 77.9,66.98 77.9,64.08 | 75.85,53.63 73.6,51.38 73.6,49.68 73.9,49.38 73.8,49.38 v73.7,49.48 | v65.55,46.68 61.3,46.68 61.1,46.88 v60.9,46.88 | v52.1,49.28 52.1,47.88 52.6,47.08 52.8,46.88 v57.8,46.88
  Top 0.256: 77.9,64.08 77.9,61.63 75.95,59.68 75.95,53.73 75.85,53.63
  Bottom 0.2: 53.62,58.18 55.65,58.18 56.15,59.03 57.5,59.03 v58.2,58.33
  Bottom 0.254: v73.7,49.48 73.7,47.98 72.6,46.68 v65.55,46.68 | v60.9,46.88 v57.8,46.88 | v52.1,49.28 LED11.AN | LED10.AN 53.62,58.18 55.6,58.18 U$26.LED_A
B_LED_K  (via drill 0.25 pad 0.65)
  Top 0.254: N5.3 74.77,67.15 74.5,66.88 v74.5,56.98 | v65.6,55.18 v61.7,55.18 | v58,49.23 57.05,47.58 v54.3,47.58
  Bottom 0.2: 59.45,49.23 v58,49.23 | U$26.LED_K 58.25,57.08 58.65,56.68 58.65,52.98 59.05,52.58 61.6,52.58 61.7,52.68
  Bottom 0.254: v74.5,56.98 74.4,56.98 72.6,55.18 v65.6,55.18 | v61.7,55.18 61.7,52.68 61.7,49.28 61.4,49.23 59.45,49.23 | v54.3,47.58 54.2,47.48 50.2,47.48 49.8,47.88 49.8,49.25 LED11.CA 48.8,49.28 48.4,49.88 48.4,56.78 49.3,57.68 49.3,58.35 LED10.CA
B_RED  (via drill 0.25 pad 0.65)
  Top 0.2: v14.95,63.68 15.15,63.68 16.8,65.33 16.8,66.98 ADC2.12
  Bottom 0.2: U$25.P$2 10.67,62.9 11.75,63.98 12.65,63.98 13.4,63.23 14.5,63.23 v14.95,63.68
BASE_LED  (via drill 0.25 pad 0.65)
  Top 0.2: U5.11 66.11,77.47 67.2,76.38 69.9,76.38 v70,76.48 | v74.7,76.98 72.55,76.98 R23.1 72.45,76.98 71.9,76.98 71.4,76.48 71.4,73.38 71.96,72.82 N5.1
  Bottom 0.2: v70,76.48 71,76.48 71.5,76.98 v74.7,76.98
BLUE_RX  (via drill 0.25 pad 0.6)
  Top 0.254: U$1.P$13 45.22,87 44.6,86.38 39.1,86.38 38.3,85.58 v38.3,83.38
  Bottom 0.254: v38.3,83.38 38.3,73.58 38.9,72.98 U$10.RX
  Bottom 0.406: U$1.P$13 U$1.P$53
BLUE_TX  (via drill 0.25 pad 0.6)
  Top 0.254: U$1.P$14 42.68,87.46 42,86.88 38.7,86.88 37.4,85.58 37.4,83.48 v37.3,83.38
  Bottom 0.254: v37.3,83.38 37.3,73.08 38.5,71.88 50.5,71.88 51,72.58 51,74.14 U$10.TX
  Bottom 0.406: U$1.P$14 U$1.P$54
CH_STAT1  (via drill 0.25 pad 0.65)
  Top 0.2: U$4.3 23.5,25.08 v24.7,25.18 | v27.2,14.08 28.1,13.18 R19.2 | U5.12 64.84,71.94 65.5,71.28 65.5,68.18 v65.6,68.02 | v65.2,35.58 61.6,35.58 60.7,36.48 59.8,36.48 v59.6,36.28 | v50.7,38.58 45.6,38.58 44.6,39.58 42.1,39.58 42.1,39.78 40.9,40.98 38.6,40.98 v38.5,41.18 | v30.7,30.58 v30.7,28.08
  Bottom 0.2: v27.2,14.08 26.7,14.08 26.5,13.88 25.4,13.88 25.2,14.08 23.8,14.08 23.5,14.38 23.5,25.08 v24.7,25.18 25.3,24.58 26.6,24.58 30.1,28.08 v30.7,28.08 | v65.6,68.02 66.34,68.02 66.8,67.6 66.8,61.68 68.7,59.78 75.1,59.78 76.5,58.38 76.5,51.68 74.3,49.48 74.3,34.88 74.2,34.78 70.2,34.78 69,35.98 68.1,35.98 68,36.08 66.7,36.08 65.9,35.28 65.5,35.28 v65.2,35.58 | v59.6,36.28 53.6,36.28 50.5,38.38 v50.7,38.58 | v38.5,41.18 39.3,40.58 39.4,38.28 39.4,34.88 34.8,30.28 31,30.28 v30.7,30.58
CH_STAT2  (via drill 0.25 pad 0.65)
  Top 0.2: U$4.4 24,22.88 25.2,22.88 | 25.2,22.88 26.2,22.88 26.2,18.13 26.7,17.28 v27,17.28 | v24,12.88 24.5,12.38 R20.2 | U5.13 v63.57,74.86 | v67.4,72.28 v69.1,72.28 | v84.2,38.28 83.8,38.28 v78.1,32.58 | v72.2,31.68 72.2,35.08 70.8,36.48 v70.6,36.28 | v65.9,39.18 60.4,39.18 59.6,38.38 51.9,38.38 50.9,39.48 46.3,39.48 v45.1,40.68 | v43,27.78 41.5,27.78 40.6,26.88 35.8,26.88 v34.6,28.08 | v25.3,23.18 25.3,22.98 25.2,22.88
  Bottom 0.2: v27,17.28 28.3,15.98 28.3,13.68 27.8,13.18 24,13.18 v24,12.88 | v63.57,74.86 64.82,74.86 v67.4,72.28 | v69.1,72.28 69.1,71.48 70.8,69.78 74.7,69.78 77.4,67.08 77.4,60.33 77.75,59.98 77.75,58.68 77.4,58.33 77.4,56.08 83,50.58 83,39.48 v84.2,38.28 | v78.1,32.58 77,32.58 76.3,31.88 72.4,31.88 v72.2,31.68 | v70.6,36.28 69,37.88 67.2,37.88 v65.9,39.18 | v45.1,40.68 45.1,28.58 44.3,27.78 v43,27.78 | v34.6,28.08 31.7,28.08 30.6,26.98 29.6,26.98 26,23.38 v25.3,23.18
ENC_L_A  (via drill 0.25 pad 0.6, 0.25 pad 0.65)
  Top 0.2: U$7.P$3 80.04,78.09 81.4,76.73 82.7,76.73 83.05,76.38 85.75,76.38 86.1,76.03 86.1,73.08 87.05,72.13 87.05,64.93 88.9,63.08 88.9,60.28 88,59.38 86.95,59.38 76.35,48.78 75.25,48.78 73.6,47.13 v73.6,46.08 | v67.4,45.13 65.35,43.13 64,41.78
  Top 0.254: v19.55,41.53 19.85,41.78 31,41.78 31.5,42.28 38.9,42.28 39.4,41.78 64,41.78 | U$21.CHA 10.6,44.08 11.3,43.38 v11.3,41.58
  Bottom 0.2: v73.6,46.08 68.8,46.08 v67.4,45.13
  Bottom 0.254: v19.55,41.53 19.3,41.68 16,41.68 15.7,41.38 14.8,41.38 14.6,41.58 v11.3,41.58
ENC_L_B  (via drill 0.25 pad 0.6, 0.25 pad 0.65)
  Top 0.2: U$7.P$2 78.77,73.35 v78.75,73.33 | v81.2,72.98 81.2,72.18 83.1,70.28 83.1,68.53 v85.4,66.23
  Top 0.254: v39,44.88 38.7,45.18 30.6,45.18 29.5,44.08 19.25,44.08 v18.85,43.68 | v40.6,44.88 41.3,44.28 43.3,44.28 v44.2,44.58 | v45.6,44.78 45.8,44.58 56.7,44.58 v57.4,45.28 | U$21.CHB 9.45,42.08 10.8,40.73 11.65,40.73 v13.4,42.48 | v59.6,45.28 66.3,45.28 67.1,46.08 68.15,46.08 69.25,44.98 v71.1,44.98 | v73.5,44.58 76.2,44.58 77.85,46.23 83.75,46.23 v84.45,46.93 | v83.7,51.33 83.7,52.43 v82.85,53.28
  Bottom 0.2: v78.75,73.33 80.85,73.33 v81.2,72.98 | v85.4,66.23 85.4,61.18 83.9,59.68 79,59.68 78.65,59.33
  Bottom 0.254: v39,44.88 v40.6,44.88 | v44.2,44.58 45.3,44.58 v45.6,44.78 | v13.4,42.48 17.65,42.48 v18.85,43.68 | v57.4,45.28 v59.6,45.28 | v71.1,44.98 73.1,44.98 v73.5,44.58 | v84.45,46.93 84.45,50.58 v83.7,51.33 | v82.85,53.28 81.9,53.28 78.65,56.53 78.65,59.33
ENC_R_A  (via drill 0.25 pad 0.65)
  Top 0.2: U$22.CHA 92.45,42.08 92.45,46.23 91.65,47.03 v90.4,47.03 | v90.35,51.03 90.35,62.43 87.45,65.33 87.45,68.93 92.15,73.63 92.15,76.13 91.45,76.83 86.4,76.83 86.05,77.18 84.4,77.18 83.85,77.73 U$7.P$6
  Bottom 0.2: v90.4,47.03 90.4,50.98 v90.35,51.03
ENC_R_B  (via drill 0.25 pad 0.65)
  Top 0.2: U$22.CHB 95.65,44.08 95.65,46.63 95,47.28 v92.85,47.28 | U$7.P$5 82.58,80.6 v82.6,80.88 | v92.2,57.03 92.2,51.28 v92.05,51.03
  Bottom 0.2: v82.6,80.88 87.5,80.88 91.95,76.23 91.95,58.18 92.2,57.98 v92.2,57.03 | v92.05,51.03 92.05,48.08 v92.85,47.28
GND  (via drill 0.25 pad 0.6, 0.25 pad 0.65, 0.35 pad 0.75)
  Top 0.2: TH1.1 39.65,37.43 39.8,37.08 | SW2.5 SW2.6 SW2.7 SW2.8 83.09,43.9 | U1.21 68.9,26.28 | PIC.2 46.5,6.68 | 46.5,6.68 46.1,6.28 39.1,6.28 38.5,5.68 38.5,4.78 U$19.1 | U$3.5-VSS 52.1,10.58 50.3,8.78 47,8.78 46.5,8.28 46.5,6.68 | 66.8,84.28 66.8,83.98 66.4,83.58 65.4,83.58 65.19,83.37 EEPROM.5 63.28,82.43 EEPROM.2 | 75.75,75.03 75.8,75.08 | N5.2 72.23,71.11 | R27.2 28.85,87.03 28.7,87.18 28.7,93.68 v29.9,94.88 | v36.4,97.38 36.4,96.68 36.5,96.58 | 62.3,2.58 67.3,3.88 66.6,5.88 70.8,7.68 v71.1,7.08 v70.5,8.38 | v80.6,98.38 82.4,97.38 84.6,95.78 v83.8,94.78 82.6,93.38 82.6,92.98 83.5,92.08 83.8,92.08 v83.9,91.98 | v91.55,32.68 90.8,31.88 89.3,31.88 88.8,31.28 88.1,30.48 88.1,29.08 84.8,25.78 v84.8,24.58 | v63.1,99.58 63.1,103.28 v63.7,103.28 | U$5.P$9 82.65,88.53 82.85,88.73 | 82.85,88.73 82.9,88.78 82.9,89.48 82.85,89.53 U$5.P$11 | 82.85,88.73 82.9,88.68 82.9,87.48 83.6,86.78 v83.6,86.48 84.1,86.18 84.6,85.68 87.95,85.68 88.45,85.18 C13.1 | U$7.P$14 77.3,83.93 v77.55,83.13 | v51,56.88 50,55.88 50,55.08 LED9.3 | U$20.3-GND 81.45,60.73 | 81.45,60.73 81.45,54.53 76.3,49.38 74.9,49.38 72.6,47.08 | 99.95,34.65 IR3.EMITTER 96.6,36.68 94.5,38.78 U$22.GND | 54.8,94.03 60.1,94.03 60.7,94.53 60.7,97.63 v60.65,97.68 | U$23.7 U$23.6 U$23.5 U$23.4 81.89,61.16 81.45,60.73 | v5,28.23 5.14,28.23 5.14,28.3 | U$25.P$5 10.67,66.71 10.8,66.58 | SW3.2 17.78,15.06 v18.15,15.53 | U$27.1 84.95,74.53 84.5,74.08 v81.2,74.08 | v60.15,48.48 60.5,48.48 60.7,48.28
  Top 0.254: U1.3 U1.2 | U1.21 65.3,26.25 65.3,27.68 63.63,27.68 U1.3 | U1.12 61.1,16.09 61.1,17.68 61.1,27.48 63.63,27.48 U1.3 | 68.9,26.28 74.8,26.28 75.2,26.68 75.2,28.48 76.1,29.38 76.1,30.98 72.7,34.38 72.7,36.58 72.2,37.08 | ADC1.4 ADC1.3 12.87,73.65 12.7,73.48 | 12.7,73.48 11.8,73.48 | 11.8,73.48 11.6,73.68 11.6,74.54 ADC1.1 11.58,76.78 | 11.58,76.78 ADC1.20 11.58,78 | 32.8,97.93 32.8,97.18 33.4,96.58 36.5,96.58 36.8,96.58 37.46,97.24 N1.2 v39,97.28 | 32.8,97.93 R9.2 | 67.7,97.38 68.8,97.38 68.8,97.34 N3.2 70.55,95.92 70.55,95.13 71.34,94.34 N6.2 | 67.7,97.38 65.75,97.38 R1.2 | 10.8,66.88 10.8,66.58 v10.8,59.68 11.58,60.46 ADC2.1 11.6,61.34 11.6,60.48 11.9,60.18 12.6,60.18 12.87,60.45 ADC2.3 ADC2.4 | v95.6,28.28 95.2,28.28 95.1,28.38 R10.2 | 32.8,97.93 32.8,97.98 27.5,97.98 24.5,96.68 v24.5,95.08 | v14.1,84.48 14.1,81.88 14.8,81.18 ADC1.15 14.8,80.17 14.8,77.48 14,76.68 11.68,76.68 11.58,76.78 | v67.7,98.18 67.7,97.38 | 10.3,71.88 9.55,71.88 C4.2 9.4,73.28 9.1,73.48 v7.7,73.48 | C3.2 13.2,72.98 12.7,73.48 | ADC2.20 10.92,67 10.8,66.88 | 10.8,66.88 10.8,67.48 10.3,67.98 10.3,71.88 | 11.8,73.48 10.9,73.48 10.3,72.88 10.3,71.88 | LED9.3 LED9.4 46.05,53.13 45.9,52.98 | R22.1 14.55,27.43 | U5.18 57.2,78.7 57.2,80.03 65.4,80.03 65.4,83.58 | U6.2 U6.1 7.14,27.64 v6.25,29.13 | 62.3,2.58 55,1.58 v55,2.38 | v36.3,5.48 33.3,6.68 IR5.EMITTER | IR6.EMITTER 5.4,33.18 6.5,30.68 4.3,29.68 5.14,28.3 7.6,24.28 10.4,24.28 10.4,22.18 12.8,19.58 13.3,20.08 v13.7,20.08 | v67.9,103.58 v66.1,105.08 | U$21.GND 13.57,46.08 VR_IR.6 | 81.45,64.31 U$20.3-GND | 54.25,84.58 54.25,83.58 U$28.GND
  Top 0.256: U$9.5-GND 54.45,93.68 54.8,94.03 | 66.8,89.48 64.4,89.48 64.25,89.63 64.25,91.83 63.95,92.13 61.9,92.13 61.35,92.68 60.6,92.68 60.1,93.18 60.1,94.03 | v62.5,97.93 62.5,98.98 v63.1,99.58
  Top 0.3: 54.25,84.58 54.85,84.58 55.75,85.48 55.75,85.93 55.85,86.03 57.3,86.03 57.75,86.48 66.75,86.48 66.8,86.43
  Top 0.305: U$4.5 25.04,23.92 | 25.04,23.92 25.4,24.28 C1.2 | 66.8,84.28 66.8,86.43 66.8,89.48 75.7,89.48 75.7,89.38 U$1.P$1 | 28.9,70.88 33,74.98 44.6,74.98 47.7,78.08 49.8,78.08 | 54.25,84.58 53.35,84.58 51.5,82.78 51.5,82.28 51,81.78 51,79.98 50.5,79.28 50,79.28 49.8,79.08 49.8,78.08 | v60.5,17.68 61.1,17.68 | R7.2 N4.2 63.64,10.54 63.6,10.58 62.4,10.58 v61.2,11.78 | 49.8,78.08 U$10.GND | 25.04,23.92 25.96,23.92 27.2,22.68 27.2,21.78 C17.2 C16.2 | C20.1 69.04,82.04 | 69.04,82.04 U4.5 | 69.04,82.04 69.49,82.04 U4.6 U4.7 70.2,82.18 70.2,83.33 | 70.55,83.79 70.3,83.79 | 70.3,83.79 70.24,83.79 U4.17 | 70.38,83.15 70.2,83.33 | C19.2 71.95,83.73 | U4.13 70.88,84.11 70.55,83.79 | U4.9 U4.10 71.95,83.73 | 71.95,83.73 70.55,83.79 | 70.2,83.33 70.3,83.79 | R22.1 14.45,26.48 14.35,26.38 14.35,22.88 14.3,22.83 14.3,22.28 14.2,22.18 14.2,21.78 14.15,21.73 14.15,20.53 v13.7,20.08
  Top 0.406: U2.12 43.02,16.09 43.7,16.78 43.7,28.68 43.6,28.78 39.34,28.78 U2.2 | U2.2 U2.3 | U2.2 43.69,28.79 v43.7,28.78 | v43.8,38.28 43.8,37.38 43.5,37.08 | R10.2 93.95,30.43 93.2,31.18 93.2,33.81 N2.2 93.83,34.55 v93.1,35.28 | U$2.- 78.9,40.19 SW2.8 | U$6.10-GND 32.9,74.88 28.9,70.88 U$6.7-GND | U$1.P$1 75.7,84.23 75.25,83.78 74.07,83.78 C19.2 | 66.8,89.48 75.6,89.48 75.7,89.38 75.7,85.58 75.8,85.48 75.8,75.08 | U$3.5-VSS 52.19,11.96 55.7,15.48 v55.7,16.58 | 14.6,27.23 R22.1 | 72.6,47.88 72.7,47.88 72.7,48.88 | POWER.1 7.92,33.91 6.5,35.33 6.5,37.18 7.1,37.78 11.05,37.78 13,35.83 14.95,35.83 15.1,35.98 | v74,74.08 73.9,73.98 73.9,72.78 72.23,71.11 | v13.7,20.08 13.8,20.18 16.3,20.18 U$17.1
  Top 0.5: C18.CATHODE 81.17,74.11 v81.2,74.08 | v74,74.08 73.45,74.08 R23.2 75.75,75.03 | 75.8,75.08 75.8,72.73 76,72.53 76,71.28 75.8,71.08 75.8,68.18 77.1,66.88 77.1,61.68 75.35,59.93 75.35,53.97 72.7,51.32 69.2,51.32 HB_R.P$8
  Top 0.6: 22.05,36.48 20.15,36.48 20.07,36.55 | 20.07,36.55 C9.2 | 20.07,36.55 19.35,35.83 17.8,35.83 15.35,35.83 15.1,35.98 VR_IR.3 VR_IR.6 15.13,44.58 18.1,44.58 18.25,44.73 C8.2
  Top 0.61: 72.4,37.08 72.2,37.08 43.5,37.08 39.8,37.08 26.5,37.08 | 26.5,37.08 25.7,37.08 25.4,36.78 C1.2 | C2.2 39.9,59.68 | 39.9,59.68 39.9,57.18 42.3,57.18 VR_L.6 43.13,57.15 44.8,55.48 44.8,54.08 45.9,52.98 v45.9,49.18 | C5.2 39.9,59.68 | HB_L.P$8 37.7,53.68 42.3,53.68 VR_L.3 42.3,49.18 | C6.2 C7.2 61.15,57.15 VR_R.6 VR_R.3 60.7,48.28 72.7,48.28 72.7,48.88 72.7,51.32 | 22.05,36.48 22.05,40.73 22.5,41.18 24.8,41.18 v26.4,39.58 | v26.4,35.98 26.4,36.98 26.5,37.08 | 42.3,49.18 v42.3,45.48 | v42.9,49.18 42.3,49.18 | 72.6,42.58 72.6,47.08 72.6,47.88 | 17.8,35.83 17.85,35.83 19.4,34.28 R18.1
  Top 0.813: U$2.- 74.87,39.71 74.85,39.73 | 74.85,39.73 74.85,38.73 73.3,37.18 72.5,37.18 72.4,37.08 | 74.85,39.73 74.85,40.93 73.4,42.38 72.8,42.38 72.6,42.58
  Bottom 0.2: v29.9,94.88 31.5,94.88 32.6,95.98 35,95.98 v36.4,97.38 | IR_B2.P4-EMITTER 46.66,106.31 46.9,106.08 50.65,106.08 51.6,106.98 IR_B3.P4-EMITTER 55.8,106.98 56.6,105.78 56.9,105.48 57.3,105.48 57.4,105.58 57.6,105.68 60.6,105.08 61.9,105.68 IR_B4.P4-EMITTER | IR4.EMITTER 71.8,5.38 v71.1,7.08 | IR2.EMITTER 97.9,75.18 97.6,75.28 96.7,77.48 98,77.98 95.9,82.38 88.9,90.88 84.1,94.98 v83.8,94.78 | v80.6,98.38 IR_B5.P4-EMITTER 78.1,99.58 76.5,96.98 69,96.98 69,99.48 68.6,99.88 63.1,99.88 v63.1,99.58 | IR3.EMITTER 97.67,34.65 96.6,33.58 92.6,33.58 v91.55,32.68 | v84.8,24.58 84.8,21.38 85.7,20.48 85.7,18.08 84.95,17.33 84.95,13.88 83.65,12.58 83.6,12.58 82.7,11.68 79.9,9.58 75.8,7.48 75,9.68 74.2,9.38 74,9.68 73.4,9.88 73.2,9.98 72.1,9.58 71.7,8.68 70.6,8.18 v70.5,8.38 | v63.7,103.28 65.9,103.28 v66.1,105.08 | v83.9,91.98 83.9,89.88 83.6,89.58 v83.6,86.48 83.6,85.18 85.6,83.28 85.6,82.18 85,81.73 84.45,81.73 83.75,82.48 77.6,82.48 77.55,82.53 v77.55,83.13 | U$18.3-GND 50.25,54.73 LED9.3 49.95,55.83 v51,56.88 | v6.25,29.13 v5,28.23 | v60.65,97.68 60.65,96.73 60.7,96.68 | v18.15,15.53 16.9,15.98 | U$26.GND 57,49.08 57.6,48.48 v60.15,48.48
  Bottom 0.254: 15.2,55.68 v10.8,59.68 | SW1.P4 93.3,24.18 94.5,25.98 94.6,26.98 v95.6,28.28 | v24.5,95.08 24.5,94.03 23.95,93.48 20.1,93.48 18.3,91.48 18.3,89.88 18.7,89.38 18.7,87.68 18,87.18 17.8,87.08 16.8,86.68 15.7,86.68 14.3,85.18 14.2,84.98 v14.1,84.48 | 67.7,96.78 v67.7,98.18 | 60.5,96.68 59.4,95.58 56.2,95.58 54.5,97.28 50.2,97.28 46.3,101.18 40.4,101.18 39,99.78 v39,97.28 | v55,2.38 48.6,2.38 48.3,2.58 47.7,2.58 46.9,1.68 46.1,1.48 40,2.58 35.6,3.88 v36.3,5.48 36.9,6.78 27.7,10.68 27.4,10.58 26.7,8.98 22.4,11.38 21.6,12.08 16.9,15.98 13.4,19.78 v13.7,20.08 | IR_B2.P4-EMITTER 42.9,106.08 42.7,105.08 39.3,104.48 35.6,103.08 35.9,102.48 30.9,100.58 | 30.9,100.58 IR8.EMITTER | IR_B1.P4-EMITTER 27.9,101.08 29.1,99.88 30.9,100.58 | IR1.EMITTER 69.6,101.38 67.8,101.38 67.8,103.58 v67.9,103.58 | v66.1,105.08 IR_B4.P4-EMITTER | v7.7,73.48 3.5,74.48 IR7.EMITTER
  Bottom 0.256: 60.5,96.68 60.7,96.68 62.25,96.68 62.4,96.83 | 62.4,96.83 62.4,97.93 v62.5,97.93 | 67.7,96.78 62.45,96.78 62.4,96.83 | 92.6,33.58 92.6,34.78 v93.1,35.28
  Bottom 0.305: v61.2,11.78 61.2,15.48 60.5,16.18 60.2,16.18 59.6,16.78
  Bottom 0.406: v43.7,28.78 43.7,38.18 v43.8,38.28 | v93.1,35.28 80.2,35.28 78.9,36.58 U$2.- | U$1.P$41 U$1.P$1 | v55.7,16.58 59.4,16.58 59.6,16.78 v60.5,17.68
  Bottom 0.5: v81.2,74.08 v74,74.08
  Bottom 0.61: v26.4,39.58 v26.4,35.98 | v42.3,45.48 42.3,38.18 43.8,38.18 v43.8,38.28 | v45.9,49.18 v42.9,49.18
  pour Bottom (isolate 0.254): 51.55,108.03 59.45,107.43 67.2,105.58 73.1,103.38 78.95,100.48 84.65,96.53 90.95,90.78 94.5,86.68 99.1,79.48 102.85,70.78 97.35,70.73 97.3,37.43 102.8,37.43 100.85,32.23 96.5,24.13 92.25,18.88 86.65,13.03 77.75,7.03 69.55,3.18 57.6,0.58 49.15,0.28 41.3,1.13 31.75,3.88 24.5,7.48 16.95,12.78 10.3,19.38 4.45,27.63 0.35,37.38 5.8,37.38 5.65,70.88 0.45,70.88 2.85,77.18 5.4,82.08 12.05,90.78 19.15,97.08 26.35,101.63 34.05,105.13 42.55,107.23 50.15,107.93
  pour Top (isolate 0.254): 0.6,70.73 6.55,83.18 16.1,94.18 26.45,101.23 40.75,106.33 51.95,107.53 66.35,105.63 78.8,99.88 87.65,92.98 96.3,83.18 102.1,71.18 96.9,71.08 97.1,37.13 102.35,37.23 99.8,30.68 92.85,19.78 85.75,13.23 77.05,7.23 67.45,3.18 55,0.88 44.75,0.83 32.4,4.33 22.25,9.08 13.65,16.08 4.95,27.23 0.65,37.03 6.5,37.03 6.3,71.38 2.65,71.28
GPIO_INT  (via drill 0.25 pad 0.65)
  Top 0.2: U1.1 62.11,30.06 v62.1,30.08 | v61.7,64.53 61.7,66.93 62.35,67.58 64.1,67.58 64.35,67.33 67.45,67.33 v68.1,67.98
  Bottom 0.2: v62.1,30.08 62.1,30.38 62.6,30.88 62.6,56.48 61.8,57.28 61.8,61.68 61.7,61.78 v61.7,64.53 | v68.1,67.98 68.1,70.78 68.3,71.08 68.3,72.28 67.8,72.78 67.8,73.38 68.5,73.88 68.55,73.93 68.55,78.58 69.6,79.63 74.75,79.63 75.25,80.13 75.25,85.13 77.2,87.08 77.2,91.68 76.7,92.18 67.7,92.18 66.1,93.98 63.55,93.98 62.7,94.83 61.55,94.83 60.45,93.73 60.45,93.68 57.3,93.68 55.8,92.18 49.17,92.18 U$1.P$52
  Bottom 0.406: U$1.P$12 U$1.P$52
ICSPCLK_2  (via drill 0.25 pad 0.65)
  Top 0.2: v80.05,85.38 U$7.P$12
  Bottom 0.2: U$27.2 87.15,75.68 86.1,76.73 82.9,76.73 80.75,78.88 77.35,78.88 76.6,79.63 76.6,84.58 77.7,85.68 79.75,85.68 v80.05,85.38
ICSPDAT_2  (via drill 0.25 pad 0.65)
  Top 0.2: U$7.P$13 78.77,85.36 78.7,85.43 77,85.43 76.85,85.28 76.85,82.23 v77.5,81.58
  Bottom 0.2: v77.5,81.58 77.5,79.88 78,79.38 80.95,79.38 83.1,77.23 86.85,77.23 87.6,76.48 88.75,76.48 89.15,76.08 U$27.3
IRPULSE_B  (via drill 0.25 pad 0.65)
  Top 0.2: U5.10 67.38,77.4 67.7,77.08 69.5,77.08 v70,77.58 | v63.8,94.68 63.8,97.93 R1.1
  Top 0.254: N3.1 63.85,99.22 R1.1
  Bottom 0.2: v70,77.58 70,78.33 70.45,78.78 75.15,78.78 76.1,79.78 76.1,84.73 78,86.63 78,91.63 78.25,91.88 78.25,92.83 77.9,93.18 67.6,93.18 66.3,94.58 63.8,94.58 v63.8,94.68
IRPULSE_F  (via drill 0.25 pad 0.65)
  Top 0.2: N1.1 36.8,99.08 v36.8,98.38 | v77.5,92.58 76.7,92.58 76.15,92.03 71,92.03 70.45,92.58 62.1,92.58 61.65,93.03 61.35,93.28 61.35,98.98 61.05,99.28 v59.7,99.28 | v69.2,73.78 66.6,73.78 66.11,73.29 U5.8
  Top 0.254: N1.1 35.89,99.12 R9.1
  Bottom 0.2: v59.7,99.28 58.6,99.28 57.6,99.18 57.3,98.98 56.8,98.98 55.6,97.78 50.5,97.78 49.7,98.48 46.5,101.68 40.1,101.68 v36.8,98.38 | v77.5,92.58 77.6,92.58 77.6,86.83 75.7,84.93 75.7,79.98 74.9,79.18 70,79.18 69.2,78.38 v69.2,73.78
IRPULSE_R  (via drill 0.25 pad 0.65)
  Top 0.2: U5.9 68.68,69.66 v68.7,69.68 | v94.2,37.38 94.2,36.69 N2.1
  Top 0.406: R10.1 95.1,35.05 N2.1
  Bottom 0.2: v68.7,69.68 69.8,69.68 70.1,69.38 74.2,69.38 77,66.58 77,60.03 77.3,59.73 77.3,58.88 77,58.58 77,55.78 82.3,50.48 82.3,38.68 83.9,37.08 93.9,37.08 v94.2,37.38
LCD_BACKLIGHT  (via drill 0.25 pad 0.6)
  Top 0.2: N4.1 59.96,12.42 v59.6,12.78
  Top 0.305: N4.1 R7.1
  Bottom 0.2: v59.6,12.78 54.4,12.78 52.5,14.68 52.5,26.48 55.1,29.08 55.1,30.68 54.2,31.58 48.2,31.58 48.1,31.68 48.1,48.48 47.9,48.68 47.9,55.38 47.9,58.98 48.4,59.48 48.4,60.38 49.7,61.68 49.7,62.23 U$1.P$70
  Bottom 0.406: U$1.P$30 U$1.P$70
LCD_RESET
  Bottom 0.2: U$3.8-RST 55.99,10.98 55,11.98 47.4,11.98 46.9,12.48 46.9,45.28 46.3,45.88 44.5,45.88 42.1,48.28 42.1,50.88 46.6,55.28 46.6,60.68 47,61.08 47.7,61.08 47.7,62.77 U$1.P$69
  Bottom 0.406: U$1.P$29 U$1.P$69
LED_GREEN  (via drill 0.25 pad 0.6)
  Top 0.254: R12.2 55.3,53.78 55,54.08 51.6,54.08 51.5,54.18 51.5,56.08 51.9,56.48 51.9,57.88 51.2,58.58 46.2,58.58 v45.65,59.13
  Bottom 0.254: v45.65,59.13 45.65,59.93 44,61.58 44,66.18 43.6,66.58 41.35,66.58 U$1.P$26
  Bottom 0.406: U$1.P$26 U$1.P$66
LED_RED  (via drill 0.25 pad 0.65)
  Top 0.2: R11.2 53.85,56.73 51.5,59.08 46.8,59.08 46.05,59.83 45.4,59.83 45.1,59.53 45.1,57.78 45.25,57.63 45.25,56.73 v45.15,56.63
  Bottom 0.2: U$1.P$65 41.95,58.48 44.05,58.48 44.4,58.13 44.9,58.13 45.1,57.93 45.1,57.78 45.25,57.63 45.25,56.73 v45.15,56.63
  Bottom 0.406: U$1.P$25 U$1.P$65
LEFTF
  Top 0.254: HB_L.P$4 33.9,60.18 31.2,60.18 31.2,64.08 27.44,64.08 U$1.P$61
  Bottom 0.406: U$1.P$21 U$1.P$61
LEFTR
  Top 0.254: U$1.P$62 29.98,48.38 33.9,48.38 HB_L.P$5
  Bottom 0.406: U$1.P$22 U$1.P$62
N$1  (via drill 0.25 pad 0.6)
  Top 0.2: U$5.P$12 82.05,90.03 81.7,89.68 81.1,89.68 80.9,89.48 v80.9,89.43 | v79.3,87.58 79.3,86.93 C12.1
  Bottom 0.2: v80.9,89.43 80.4,89.18 79.3,88.08 v79.3,87.58
N$2
  Top 0.406: U$3.3-CAPP 49.65,12.07 C15.2
N$3
  Bottom 0.406: U$1.P$43 U$1.P$3
N$4
  Bottom 0.406: U$1.P$44 U$1.P$4
N$5
  Top 0.406: C15.1 47.95,11 U$3.2-CAPN
N$6  (via drill 0.25 pad 0.65)
  Top 0.254: N6.3 75.42,94.61 v75.55,94.48 | v91.95,79.58 91.95,78.33 U$24.-
  Bottom 0.254: v75.55,94.48 75.65,94.38 81.5,94.38 83.15,92.78 83.3,92.63 84.1,92.63 84.5,92.23 84.5,91.73 84.35,91.58 84.35,87.18 v91.95,79.58
N$7  (via drill 0.25 pad 0.6)
  Top 0.305: v71.3,10.78 N4.3
  Bottom 0.2: U$3.LED-K 78.95,25.93
  Bottom 0.305: 78.95,25.93 76.3,23.28 76.3,12.58 74.5,10.78 v71.3,10.78
N$8
  Top 0.406: C14.1 45.41,12.28 U$3.1-VOUT
N$9
  Top 0.406: U$6.8-ANT 31.3,70.88 28.5,68.18 23.55,68.18 21.75,66.38 U$8.ANT
N$10  (via drill 0.25 pad 0.6)
  Top 0.305: v80.9,11.98 R8.2
  Bottom 0.305: 78.95,15.93 U$3.LED-A 78.95,13.93 v80.9,11.98
N$11
  Top 0.254: LED9.1 R11.1
N$13  (via drill 0.25 pad 0.65)
  Top 0.254: U$4.6 24.49,26.37 24.3,26.18 22.7,26.18 22.6,26.28 22.6,26.58 22.4,26.78 22.3,26.78 v21.4,27.58 | R18.2 19.45,30.08 20.9,30.08 21,29.98 v21,29.38
  Bottom 0.254: v21.4,27.58 21.4,28.98 v21,29.38
N$14  (via drill 0.25 pad 0.65, 0.35 pad 0.75)
  Top 0.2: U$14.AN 34.95,9.28 v33,9.28 | v28,24.38 27.1,25.28 U$11.P$3 | v33.6,15.43 v33.6,18.78
  Top 0.254: U$13.AN U$12.AN U$14.AN | U$15.5 17.35,27.58 17.35,27.23 17.2,27.08 17.2,26.38 17.6,25.98 19.4,25.98 v19.7,25.68 20.3,25.68 21.15,24.83 R28.2
  Top 0.305: U$15.1 20.38,26.35 v19.7,25.68 | v27.2,30.18 27.2,27.78 U$11.P$3
  Bottom 0.2: v33.6,18.78 v28,24.38 | v33,9.28 33,14.78 v33.6,15.43
  Bottom 0.305: v19.7,25.68 19.7,29.28 20.7,30.28 27.1,30.28 v27.2,30.18
N$16
  Top 0.254: R29.1 89.65,80.83 U$24.+
N$18
  Bottom 0.406: U$1.P$58 U$1.P$18
N$19
  Bottom 0.406: U$1.P$59 U$1.P$19
N$20
  Bottom 0.406: U$1.P$60 U$1.P$20
N$21
  Top 0.2: U$12.CA 37.7,11.08 37.6,10.98 33.2,10.98 31.5,11.58 29.9,11.58 R19.1
N$22
  Top 0.406: USB_CHARGE.1 73.16,68.38 U$1.P$39
  Bottom 0.406: U$1.P$39 U$1.P$79
N$23
  Bottom 0.406: U$1.P$38 U$1.P$78
N$24
  Bottom 0.406: U$1.P$37 U$1.P$77
N$25
  Bottom 0.406: U$1.P$36 U$1.P$76
N$26
  Bottom 0.406: U$1.P$35 U$1.P$75
N$27
  Bottom 0.406: U$1.P$34 U$1.P$74
N$28
  Bottom 0.406: U$1.P$33 U$1.P$73
N$29
  Bottom 0.406: U$1.P$32 U$1.P$72
N$30
  Bottom 0.406: U$1.P$31 U$1.P$71
N$31
  Top 0.254: R12.1 53.65,50.83 53.1,51.38 53.1,53.08 LED9.2
N$32
  Top 0.2: U$13.CA 40.5,10.88 40.15,10.58 32.9,10.58 31.4,11.18 26.8,11.18 26.7,11.28 R20.1
N$33
  Top 0.2: U$14.CA 35,12.15 35,12.48 R21.1
N$34
  Top 0.2: U$5.P$8 81.75,87.68 C12.2
N$35  (via drill 0.25 pad 0.65)
  Top 0.2: U$5.P$10 81.8,89.03 v81.6,88.83 | v84.8,82.68 85.75,82.68 86.05,82.98 87.15,82.98 87.3,83.13 87.3,84.08 C13.2 86.7,84.73
  Bottom 0.2: v81.6,88.83 81.6,86.13 v84.8,82.68
N$36  (via drill 0.25 pad 0.65)
  Top 0.2: U$4.8 v23.5,26.88 | v30.8,13.38 31.2,12.98 R21.2
  Bottom 0.2: v23.5,26.88 21.6,26.88 21.2,26.48 21.2,24.78 22.8,23.18 22.8,17.58 21.4,16.18 21.4,14.08 23,12.48 26.2,10.48 26.8,11.58 27.5,11.88 27.8,11.88 29,11.38 30.8,10.58 v30.8,13.38
N$37
  Top 0.61: U$17.2 18.35,21.23 U$16.P$1
N$38  (via drill 0.25 pad 0.65, 0.35 pad 0.75)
